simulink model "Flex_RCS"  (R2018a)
settings: Solver=ode4  StartTime=0.0  StopTime=600  FixedStep=Ts  RelTol=1e-3  EnableMultiTasking=on
InitFcn:
  | runf
StopFcn:
  | plf
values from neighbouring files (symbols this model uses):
  d2r = pi/180    (= 0.0174532925199)    [runf.m]    (also in run.m; orbitic.m; Quan.m)
  nt = 7    [runf.m]    (also in run.m)
  Ts = 0.0005    [runf.m]    (also in run.m = 0.001)
undefined symbols (not defined in the file or in its folder): Avf, Bvf, Cvf, Dvf, Phase_Plane
libraries: simulink x1

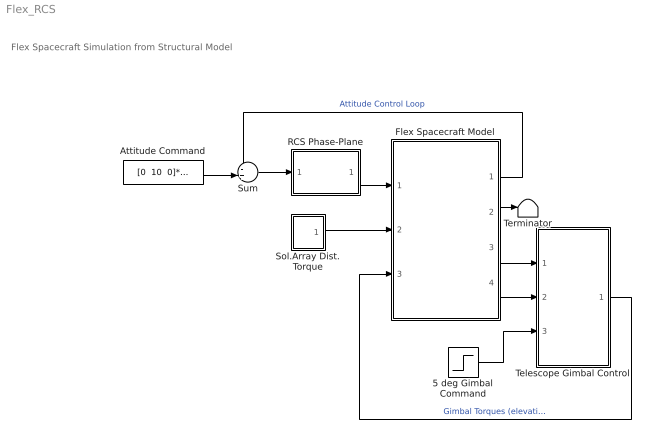
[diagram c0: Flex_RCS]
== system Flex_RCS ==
  note: Flex Spacecraft Simulation from Structural Model
  5 deg Gimbal Command : Step  Time=20  After=[5, 5]*d2r  SampleTime=0
  Attitude Command : Constant  Value="[0  10  0]*d2r"
  Flex Spacecraft Model : Subsystem
  RCS Phase-Plane : Subsystem
  Sol.Array Dist. Torque : Subsystem
  Sum : Sum  Inputs=-+|
  Telescope Gimbal Control : Subsystem
  Terminator : Terminator
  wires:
  Flex Spacecraft Model/1(att-flx) -> Sum/1  "Attitude Control Loop"
  Flex Spacecraft Model/3(Gimb) -> Telescope Gimbal Control/1(Gimb)
  Flex Spacecraft Model/4(Gdot) -> Telescope Gimbal Control/2(Grate)
  Telescope Gimbal Control/1(GTrq) -> Flex Spacecraft Model/3(Tgmb)  "Gimbal Torques (elevation, zimuth)"
  Flex Spacecraft Model/2(wb-flx) -> Terminator/1
  Attitude Command/1 -> Sum/2
  Sum/1 -> RCS Phase-Plane/1(atter)
  Sol.Array Dist. Torque/1(Tsa) -> Flex Spacecraft Model/2(Tsolar)
  5 deg Gimbal Command/1 -> Telescope Gimbal Control/3(Cmd)
  RCS Phase-Plane/1(f(nt)) -> Flex Spacecraft Model/1(Frcs)

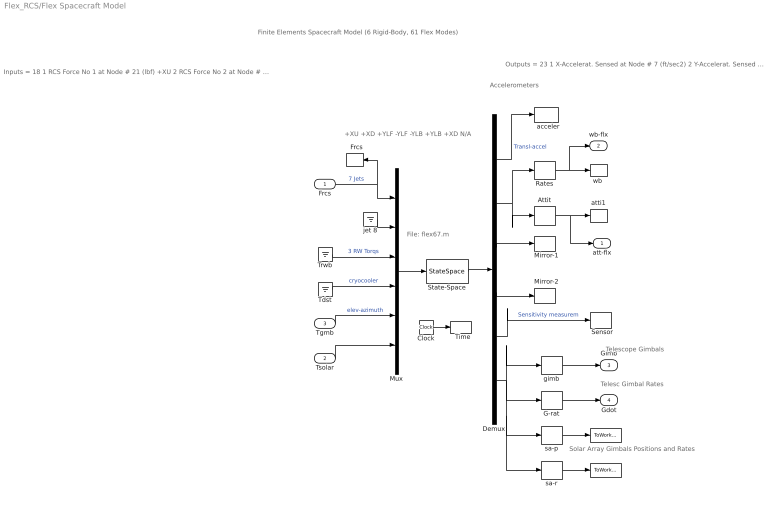
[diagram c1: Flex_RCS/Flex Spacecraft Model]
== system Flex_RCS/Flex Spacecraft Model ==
  note: Accelerometers
  note: +XU +XD +YLF -YLF -YLB +YLB +XD N/A
  note: Outputs = 23 1 X-Accelerat. Sensed at Node # 7 (ft/sec2) 2 Y-Accelerat. Sensed at Node # 7 (ft/sec2) 3 X-Rot. Rate Sensed at Node # 6 (radian) 4 Y-Rot. Rate Sensed at Node # 6 (radian) 5 Z-Rot. Rate Sensed at Node # 6 (radian) 6 X-Rotation Sensed at Node # 6 (radian) 7 Y-Rotation Sensed at Node # 6 (radian) 8 Z-Rotation Sensed at Node # 6 (radian) 9 Y-Rotation Mirror at Node # 9 (radian) 10 Z-Rotation Mirror at Node # 9 (radian) 11 Y-Rotation Instrum-2 Node # 10 (radian) 12 Z-Rotation Instrum-2 Node # 10 (radian) 13 X-Rotation Instrum-3 Node # 11 (radian) 14 Y-Rotation Instrum-4 Node # 12 (radian) 15 Z-Rotation Instrum-5 Node # 13 (radian) 16 Rotation Angle at Elevati Gimbal No 1 17 Rotation Rate at Elevati Gimbal No 1 18 Rotation Angle at Azimuth Gimbal No 2 19 Rotation Rate at Azimuth Gimbal No 2 20 Rotation Angle at Rght SA Gimbal No 3 21 Rotation Rate at Rght SA Gimbal No 3 22 Rotation Angle at Left SA Gimbal No 4 23 Rotation Rate at Left SA Gimbal No 4
  note: Inputs = 18 1 RCS Force No 1 at Node # 21 (lbf) +XU 2 RCS Force No 2 at Node # 22 (lbf) +XD 3 RCS Force No 3 at Node # 23 (lbf) +YLF 4 RCS Force No 4 at Node # 24 (lbf) -YLF 5 RCS Force No 5 at Node # 25 (lbf) -YLB 6 RCS Force No 6 at Node # 26 (lbf) +YLB 7 RCS Force No 7 at Node # 27 (lbf) +XD 8 RCS Force No 8 at Node # 28 (lbf) +X n/a 9 RW Torque No 1 at Node # 17 (ft-lb) roll 10 RW Torque No 2 at Node # 18 (ft-lb) ptch 11 RW Torque No 3 at Node # 19 (ft-lb) yaw 12 Dist Trque No 4 at Node # 8 (ft-lb) roll 13 Dist Trque No 5 at Node # 8 (ft-lb) ptch 14 Dist Trque No 6 at Node # 8 (ft-lb) yaw 15 Elevation Trqu at Gimbal No 1 (ft-lb) 16 Azimuth Torque at Gimbal No 2 (ft-lb) 17 Rght SA Torque at Gimbal No 3 (ft-lb) 18 Left SA Torque at Gimbal No 4 (ft-lb)
  note: Finite Elements Spacecraft Model (6 Rigid-Body, 61 Flex Modes)
  note: Telescope Gimbals
  note: Telesc Gimbal Rates
  note: File: flex67.m
  note: Solar Array Gimbals Positions and Rates
  Frcs : Inport
  Tsolar : Inport  Port=2
  Tgmb : Inport  Port=3
  " " : ToWorkspace  VariableName=SA_pos  SampleTime=-1
  "   " : ToWorkspace  VariableName=SA_rate  SampleTime=-1
  "  Frcs" : ToWorkspace  VariableName=Frcs  SampleTime=-1
  "  Mirror-1" : ToWorkspace  VariableName=Mir1  SampleTime=-1
  "  Mirror-2" : ToWorkspace  VariableName=Mir2  SampleTime=-1
  "  Sensor" : ToWorkspace  VariableName=Sens  SampleTime=-1
  "  Time" : ToWorkspace  VariableName=time  SampleTime=-1
  "  acceler" : ToWorkspace  VariableName=accel  SampleTime=-1
  Attit : Selector  InputPortWidth=6  IndexOptions=Index vector (dialog)  Indices=[4:6]  OutputSizes=1
  Clock : Clock
  Demux : Demux  Outputs="[2, 6, 2,2,3,  8]"
  G-rat : Selector  InputPortWidth=8  IndexOptions=Index vector (dialog)  Indices="[2  4]"  OutputSizes=1
  Mux : Mux  Inputs=[7,1,3,3,2,2]
  Rates : Selector  InputPortWidth=6  IndexOptions=Index vector (dialog)  Indices=[1:3]  OutputSizes=1
  State-Space : StateSpace  A=Avf  B=Bvf  C=Cvf  D=Dvf  InitialCondition=0
  Tdst : Ground
  Trwb : Ground
  atti1 : ToWorkspace  VariableName=atti  SampleTime=-1
  gimb : Selector  InputPortWidth=8  IndexOptions=Index vector (dialog)  Indices=[1 3]  OutputSizes=1
  jet 8 : Ground
  sa-p : Selector  InputPortWidth=8  IndexOptions=Index vector (dialog)  Indices=[5, 7]  OutputSizes=1
  sa-r : Selector  InputPortWidth=8  IndexOptions=Index vector (dialog)  Indices=[6, 8]  OutputSizes=1
  "wb " : ToWorkspace  VariableName=wb  SampleTime=-1
  att-flx : Outport
  wb-flx : Outport  Port=2
  Gimb : Outport  Port=3
  Gdot : Outport  Port=4
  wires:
  Demux/4 -> "  Mirror-2"/1
  Demux/3 -> "  Mirror-1"/1
  Demux/5 -> "  Sensor"/1  "Sensitivity measurem"
  Tsolar/1 -> Mux/6
  Tdst/1 -> Mux/4  "cryocooler"
  Trwb/1 -> Mux/3  "3 RW Torqs"
  jet 8/1 -> Mux/2
  Frcs/1 -> Mux/1, "  Frcs"/1  "7 Jets"
  Mux/1 -> State-Space/1
  Rates/1 -> wb-flx/1, "wb "/1
  Attit/1 -> atti1/1, att-flx/1
  State-Space/1 -> Demux/1
  Demux/1 -> "  acceler"/1  "Transl-accel"
  gimb/1 -> Gimb/1
  G-rat/1 -> Gdot/1
  Tgmb/1 -> Mux/5  "elev-azimuth"
  Clock/1 -> "  Time"/1
  Demux/2 -> Attit/1, Rates/1
  sa-r/1 -> "   "/1
  sa-p/1 -> " "/1
  Demux/6 -> sa-r/1, sa-p/1, G-rat/1, gimb/1

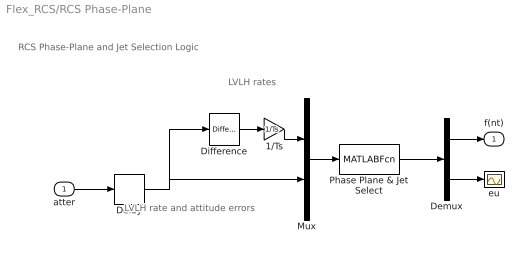
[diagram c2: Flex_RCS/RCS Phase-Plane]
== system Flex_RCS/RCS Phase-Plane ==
  note: RCS Phase-Plane and Jet Selection Logic
  note: LVLH rate and attitude errors
  note: LVLH rates
  atter : Inport
  1/Ts : Gain  Gain=1/Ts
  Delay : Delay  DelayLength=1  InputProcessing=Inherited
  Demux : Demux  Outputs=[nt, 3]
  Difference : simulink/Discrete/Difference  ICPrevInput=0.0  InputProcessing=Inherited  OutMin=[]  OutMax=[]  OutDataType=sfix(16)  OutScaling=2^-10  DoSatur=off
  Mux : Mux  Inputs="[3  3]"
  Phase Plane & Jet Select : MATLABFcn  MATLABFcn=Phase_Plane( u(1:3), u(4:6) )  OutputDimensions=nt + 3
  eu : Scope
  f(nt) : Outport
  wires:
  atter/1 -> Delay/1
  1/Ts/1 -> Mux/1
  Demux/2 -> eu/1
  Demux/1 -> f(nt)/1
  Phase Plane & Jet Select/1 -> Demux/1
  Mux/1 -> Phase Plane & Jet Select/1
  Difference/1 -> 1/Ts/1
  Delay/1 -> Mux/2, Difference/1

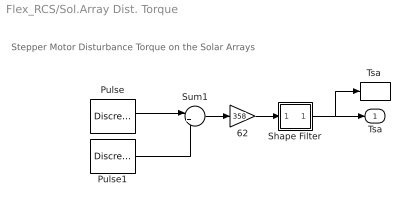
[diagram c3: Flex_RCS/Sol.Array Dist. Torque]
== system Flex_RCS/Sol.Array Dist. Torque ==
  note: Stepper Motor Disturbance Torque on the Solar Arrays
  62 : Gain  Gain=358
  Pulse : DiscretePulseGenerator  PulseType=Time based  Amplitude="0.001*[1  1]"  Period="0.5*[1  1]"  PulseWidth="4*[1  1]"
  Pulse1 : DiscretePulseGenerator  PulseType=Time based  Amplitude="-0.001*[1  1]"  Period="0.5*[1  1]"  PulseWidth="4*[1  1]"  PhaseDelay="0.25*[1  1]"
  Shape Filter : Subsystem
  Sum1 : Sum  Inputs=|++
  "Tsa " : ToWorkspace  VariableName=Tsa  SampleTime=-1
  Tsa : Outport
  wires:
  Sum1/1 -> 62/1
  62/1 -> Shape Filter/1(I)
  Pulse1/1 -> Sum1/2
  Pulse/1 -> Sum1/1
  Shape Filter/1(O) -> "Tsa "/1, Tsa/1

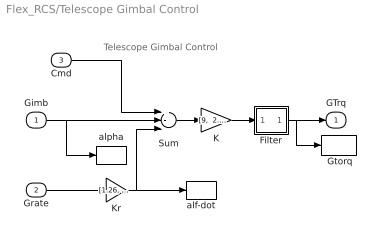
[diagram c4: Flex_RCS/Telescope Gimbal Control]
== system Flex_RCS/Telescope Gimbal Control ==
  note: Telescope Gimbal Control
  Gimb : Inport
  Grate : Inport  Port=2
  Cmd : Inport  Port=3
  " Gtorq" : ToWorkspace  VariableName=Gtrq  SampleTime=-1
  Filter : Subsystem
  K : Gain  Gain="[9,  2.85]"
  Kr : Gain  Gain="[1.26,  1.14]"
  Sum : Sum  Inputs=+--
  alf-dot : ToWorkspace  VariableName=Grate  SampleTime=-1
  alpha : ToWorkspace  VariableName=gimb  SampleTime=-1
  GTrq : Outport
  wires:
  Sum/1 -> K/1
  Gimb/1 -> Sum/2, alpha/1
  Grate/1 -> Kr/1
  K/1 -> Filter/1(I)
  Kr/1 -> Sum/3, alf-dot/1
  Cmd/1 -> Sum/1
  Filter/1(O) -> GTrq/1, " Gtorq"/1

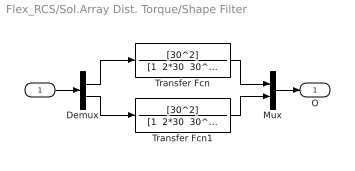
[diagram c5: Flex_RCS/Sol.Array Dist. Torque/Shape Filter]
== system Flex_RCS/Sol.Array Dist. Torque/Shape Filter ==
  I : Inport
  Demux : Demux  Outputs=2
  Mux : Mux  Inputs=2
  Transfer Fcn : TransferFcn  Numerator=[30^2]  Denominator="[1  2*30  30^2]"
  Transfer Fcn1 : TransferFcn  Numerator=[30^2]  Denominator="[1  2*30  30^2]"
  O : Outport
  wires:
  Mux/1 -> O/1
  I/1 -> Demux/1
  Transfer Fcn1/1 -> Mux/2
  Transfer Fcn/1 -> Mux/1
  Demux/1 -> Transfer Fcn/1
  Demux/2 -> Transfer Fcn1/1

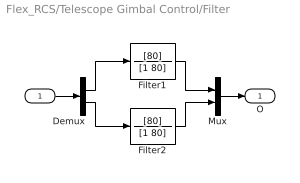
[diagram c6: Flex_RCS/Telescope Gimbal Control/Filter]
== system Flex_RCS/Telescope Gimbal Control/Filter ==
  I : Inport
  Demux : Demux  Outputs=2
  Filter1 : TransferFcn  Numerator=[80]  Denominator=[1 80]
  Filter2 : TransferFcn  Numerator=[80]  Denominator=[1 80]
  Mux : Mux  Inputs=2
  O : Outport
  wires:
  Mux/1 -> O/1
  I/1 -> Demux/1
  Demux/2 -> Filter2/1
  Demux/1 -> Filter1/1
  Filter2/1 -> Mux/2
  Filter1/1 -> Mux/1
